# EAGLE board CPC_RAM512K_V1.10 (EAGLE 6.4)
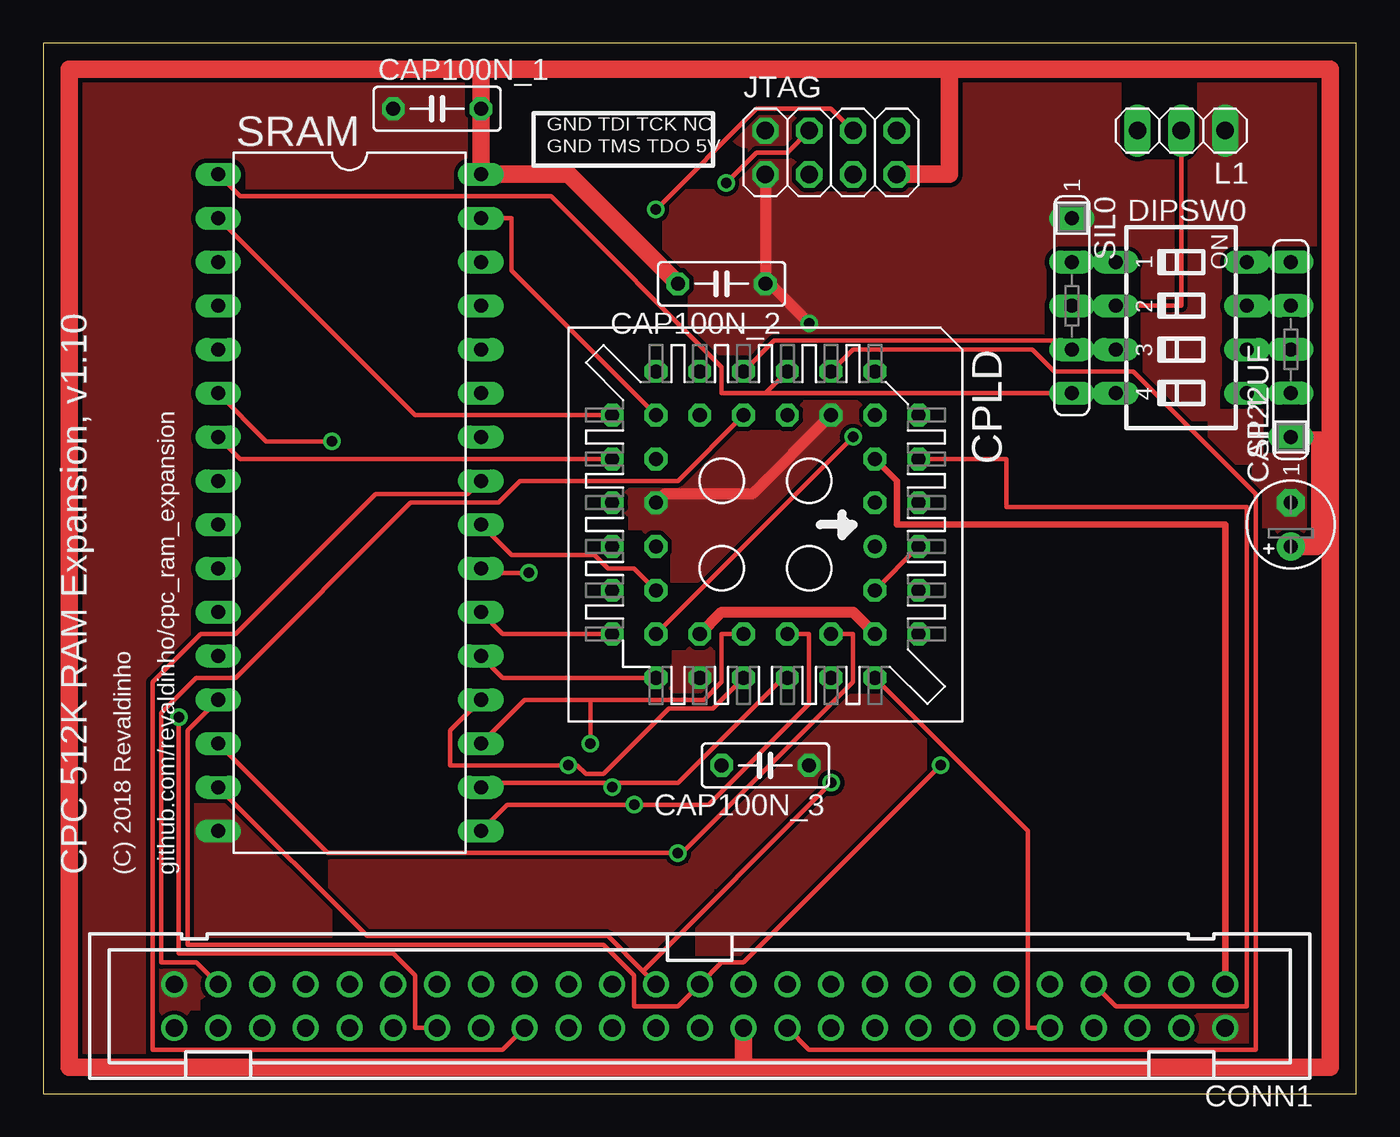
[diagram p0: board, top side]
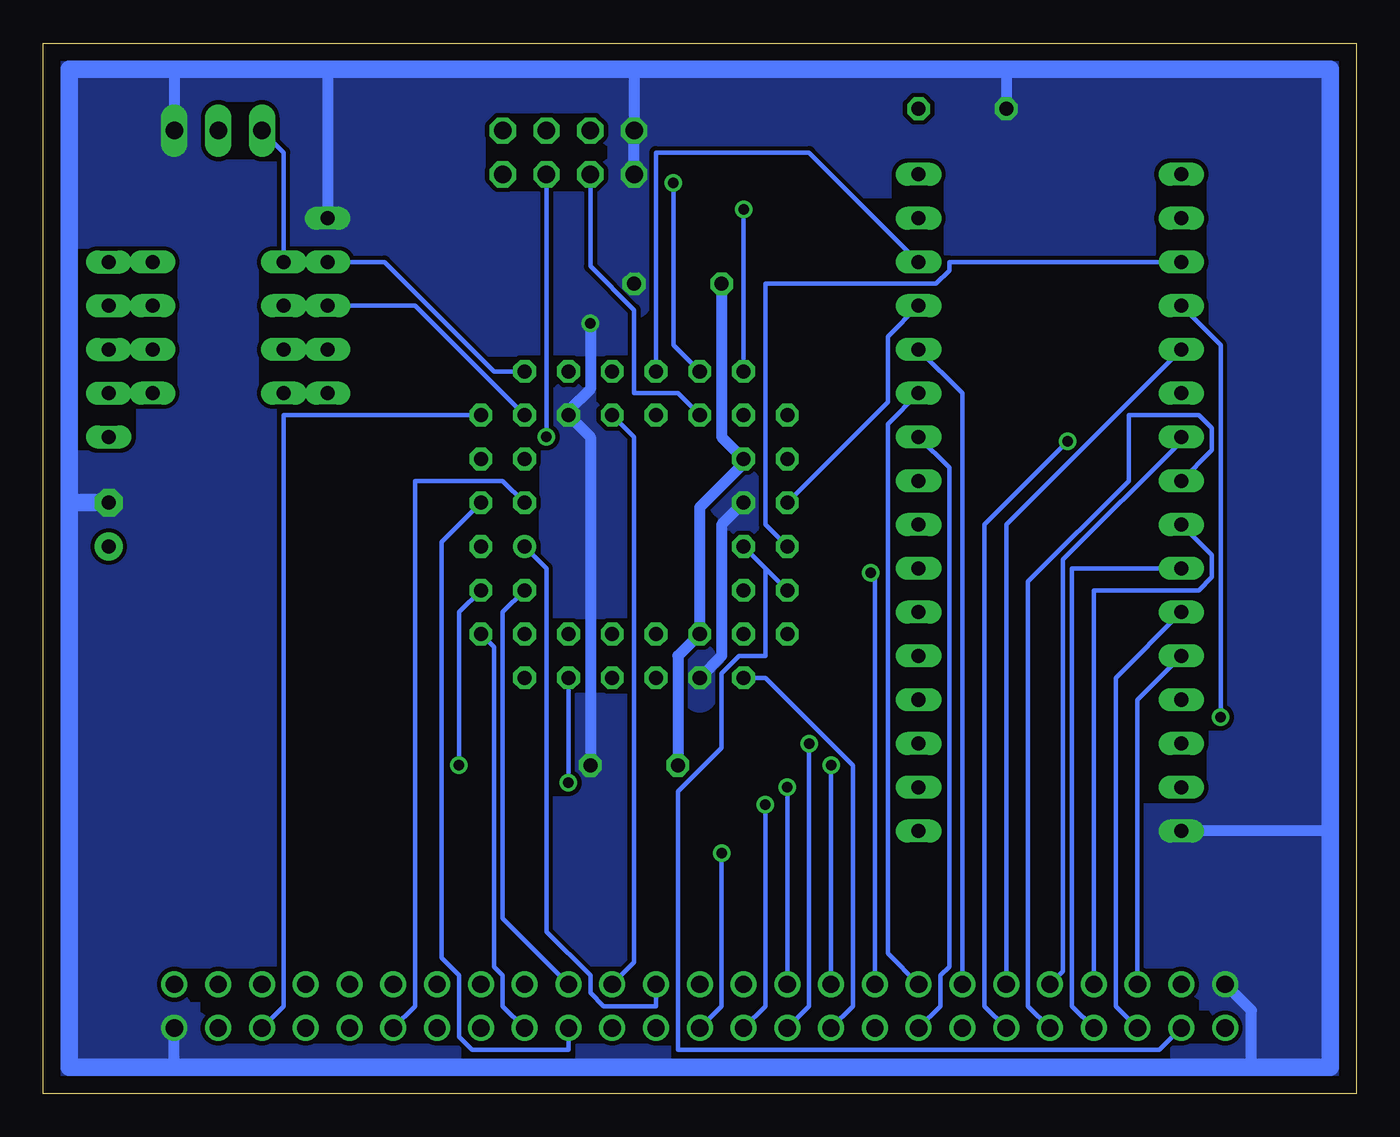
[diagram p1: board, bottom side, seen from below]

Size 76.2 x 60.96 mm. Coordinates in mm from the lower left corner, seen from the top.
Outline: 0,0 76.2,0 76.2,60.96 0,60.96 0,0
Copper layers (1*16): Top 0.035mm / dielectric 1.5mm / Bottom 0.035mm
Design rules "default": minimum track width 10mil, minimum drill 24mil, track to track 8mil, track to pad 8mil, pad to pad 8mil, via to via 8mil, smd to smd 8mil, copper to edge 40mil, drill to drill 8mil, minimum pad ring 10mil, minimum via ring 8mil, stop-mask expansion 4mil, vias tented up to drill 0mil, thermal gap 10mil
Net classes: 0 signal: width 0.254 mm, clearance 0.254 mm; 1 supply: width 0.635 mm, clearance 0.254 mm

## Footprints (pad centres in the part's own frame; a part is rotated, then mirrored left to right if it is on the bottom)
E2,5-5 = drill 0.813 pad 1.6: + -1.27,0 | drill 0.813 pad 1.6 octagon: - 1.27,0
C050-025X075 = drill 0.813 octagon: 1 -2.54,0; 2 2.54,0
PAK100/2500-50 = drill 1 pad 1.422: 1 -30.48,-1.27; 2 -30.48,1.27; 3 -27.94,-1.27; 4 -27.94,1.27; 5 -25.4,-1.27; 6 -25.4,1.27; 7 -22.86,-1.27; 8 -22.86,1.27; 9 -20.32,-1.27; 10 -20.32,1.27; 11 -17.78,-1.27; 12 -17.78,1.27; 13 -15.24,-1.27; 14 -15.24,1.27; 15 -12.7,-1.27; 16 -12.7,1.27; 17 -10.16,-1.27; 18 -10.16,1.27; 19 -7.62,-1.27; 20 -7.62,1.27; 21 -5.08,-1.27; 22 -5.08,1.27; 23 -2.54,-1.27; 24 -2.54,1.27; 25 0,-1.27; 26 0,1.27; 27 2.54,-1.27; 28 2.54,1.27; 29 5.08,-1.27; 30 5.08,1.27; 31 7.62,-1.27; 32 7.62,1.27; 33 10.16,-1.27; 34 10.16,1.27; 35 12.7,-1.27; 36 12.7,1.27; 37 15.24,-1.27; 38 15.24,1.27; 39 17.78,-1.27; 40 17.78,1.27; 41 20.32,-1.27; 42 20.32,1.27; 43 22.86,-1.27; 44 22.86,1.27; 45 25.4,-1.27; 46 25.4,1.27; 47 27.94,-1.27; 48 27.94,1.27; 49 30.48,-1.27; 50 30.48,1.27
PLCC-S44-SOCKET = drill 0.813: 1 1.27,6.35 | drill 0.813 octagon: 2 -1.27,8.89; 3 -1.27,6.35; 4 -3.81,8.89; 5 -3.81,6.35; 6 -6.35,8.89; 7 -8.89,6.35; 8 -6.35,6.35; 9 -8.89,3.81; 10 -6.35,3.81; 11 -8.89,1.27; 12 -6.35,1.27; 13 -8.89,-1.27; 14 -6.35,-1.27; 15 -8.89,-3.81; 16 -6.35,-3.81; 17 -8.89,-6.35; 18 -6.35,-8.89; 19 -6.35,-6.35; 20 -3.81,-8.89; 21 -3.81,-6.35; 22 -1.27,-8.89; 23 -1.27,-6.35; 24 1.27,-8.89; 25 1.27,-6.35; 26 3.81,-8.89; 27 3.81,-6.35; 28 6.35,-8.89; 29 8.89,-6.35; 30 6.35,-6.35; 31 8.89,-3.81; 32 6.35,-3.81; 33 8.89,-1.27; 34 6.35,-1.27; 35 8.89,1.27; 36 6.35,1.27; 37 8.89,3.81; 38 6.35,3.81; 39 8.89,6.35; 40 6.35,8.89; 41 6.35,6.35; 42 3.81,8.89; 43 3.81,6.35; 44 1.27,8.89
SD4-04 = drill 0.813 long: 1 -3.81,-3.81; 2 -1.27,-3.81; 3 1.27,-3.81; 4 3.81,-3.81; 5 3.81,3.81; 6 1.27,3.81; 7 -1.27,3.81; 8 -3.81,3.81
2X04 = drill 1.016 octagon: 1 -3.81,-1.27; 2 -3.81,1.27; 3 -1.27,-1.27; 4 -1.27,1.27; 5 1.27,-1.27; 6 1.27,1.27; 7 3.81,-1.27; 8 3.81,1.27
1X03 = drill 1.016 long: 1 -2.54,0; 2 0,0; 3 2.54,0
SIL5 = drill 0.813 long: 1 -5.08,0; 2 -2.54,0; 3 0,0; 4 2.54,0; 5 5.08,0
DIL32 = drill 0.813 long: 1 -19.05,-7.62; 2 -16.51,-7.62; 3 -13.97,-7.62; 4 -11.43,-7.62; 5 -8.89,-7.62; 6 -6.35,-7.62; 7 -3.81,-7.62; 8 -1.27,-7.62; 9 1.27,-7.62; 10 3.81,-7.62; 11 6.35,-7.62; 12 8.89,-7.62; 13 11.43,-7.62; 14 13.97,-7.62; 15 16.51,-7.62; 16 19.05,-7.62; 17 19.05,7.62; 18 16.51,7.62; 19 13.97,7.62; 20 11.43,7.62; 21 8.89,7.62; 22 6.35,7.62; 23 3.81,7.62; 24 1.27,7.62; 25 -1.27,7.62; 26 -3.81,7.62; 27 -6.35,7.62; 28 -8.89,7.62; 29 -11.43,7.62; 30 -13.97,7.62; 31 -16.51,7.62; 32 -19.05,7.62

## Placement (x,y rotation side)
CAP22UF  [E2,5-5]  72.39,33.02 90 top
CAP100N_1  [C050-025X075]  22.86,57.15 0 top
CAP100N_2  [C050-025X075]  39.37,46.99 180 top
CAP100N_3  [C050-025X075]  41.91,19.05 180 top
CONN1  [PAK100/2500-50]  38.1,5.08 180 top
CPLD  [PLCC-S44-SOCKET]  41.91,33.02 270 top
DIPSW0  [SD4-04]  66.04,44.45 270 top
JTAG  [2X04]  45.72,54.61 0 top
L1  [1X03]  66.04,55.88 180 top
SIL0  [SIL5]  59.69,45.72 270 top
SIL1  [SIL5]  72.39,43.18 90 top
SRAM  [DIL32]  17.78,34.29 270 top

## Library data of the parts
CAP22UF CAP100N_1-CAP100N_3 = resistor
CONN1 = con-3m
CPLD SRAM = ic-package
DIPSW0 = switch-dil
JTAG L1 = pinhead
SIL0 SIL1 = resistor-sil

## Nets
A0: CONN1.33 SRAM.23
A1: CONN1.34 SRAM.25
A2: CONN1.35 SRAM.27
A3: CONN1.36 SRAM.26
A4: CONN1.37 SRAM.28
A5: CONN1.38 SRAM.4
A6: CONN1.39 SRAM.5
A7: CONN1.40 SRAM.6
A8: CONN1.41 CPLD.20 SRAM.7
A9: CONN1.42 SRAM.8
A10: CONN1.43 SRAM.9
A11: CONN1.44 SRAM.10
A12: CONN1.45 SRAM.12
A13: CONN1.46 SRAM.11
A14: CONN1.47 CPLD.14
A15: CONN1.48 CPLD.25 CPLD.26
BUSACK_B: CONN1.13
BUSRESET_B: CONN1.11
BUSRQ_B: CONN1.14
CLK: CONN1.1 CPLD.5
CURSOR: CONN1.5
D0: CONN1.25 CPLD.42 SRAM.13
D1: CONN1.26 CPLD.38 SRAM.14
D2: CONN1.27 CPLD.37 SRAM.15
D3: CONN1.28 CPLD.36 SRAM.17
D4: CONN1.29 CPLD.35 SRAM.18
D5: CONN1.30 CPLD.34 SRAM.19
D6: CONN1.31 CPLD.33 SRAM.20
D7: CONN1.32 CPLD.29 SRAM.21
DIP0: CPLD.7 DIPSW0.1 L1.3 SIL0.2
DIP0_PU: DIPSW0.8 SIL1.5
DIP1: CPLD.8 DIPSW0.2 L1.2 SIL0.3
DIP1_PU: DIPSW0.7 SIL1.4
DIP2_PU: DIPSW0.6 SIL1.3
DIP3_PU: DIPSW0.5 SIL1.2
EXP_B: CONN1.3
HALT_B: CONN1.17
HIADR0: CPLD.24 SRAM.3
HIADR1: CPLD.19 SRAM.31
HIADR2: CPLD.18 SRAM.2
HIADR3: CPLD.13 DIPSW0.3 SIL0.4 SRAM.30
HIADR4: CPLD.11 DIPSW0.4 SIL0.5 SRAM.1
INT_B: CONN1.16
IOREQ_B: CONN1.20 CPLD.2
LPEN: CONN1.4
M1_B: CONN1.22 CPLD.9
MREQ_B: CONN1.23 CPLD.1
NMI_B: CONN1.15
RAMCS_B: CPLD.28 SRAM.22
RAMDIS: CONN1.6 CPLD.6
RAMOE_B: CPLD.27 SRAM.24
RAMRD_B: CONN1.7 CPLD.4
RAMWE_B: CPLD.22 SRAM.29
RD_B: CONN1.19 CPLD.43 CPLD.44
READY: CONN1.12 CPLD.3
RESET_B: CONN1.10 CPLD.39
RFSH_B: CONN1.21 CPLD.12
ROMDIS: CONN1.8
ROMEN_B: CONN1.9
SOUND: CONN1.50
TCK: CPLD.17 JTAG.6
TDI: CPLD.15 JTAG.4
TDO: CPLD.30 JTAG.5
TMS: CPLD.16 JTAG.3
VDD [supply]: CAP22UF.+ CAP100N_1.2 CAP100N_2.2 CAP100N_3.2 CONN1.24 CPLD.21 CPLD.32 CPLD.41 JTAG.7 SIL1.1 SRAM.32
VSS [supply]: CAP22UF.- CAP100N_1.1 CAP100N_2.1 CAP100N_3.1 CONN1.2 CONN1.49 CPLD.10 CPLD.23 CPLD.31 JTAG.1 JTAG.2 L1.1 SIL0.1 SRAM.16
WR_B: CONN1.18 CPLD.40

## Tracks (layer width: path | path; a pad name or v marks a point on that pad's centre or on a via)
A0  (via drill 0.61)
  Top 0.254: SRAM.23 25.65,30.23 v28.19,30.23
  Bottom 0.254: v28.19,30.23 27.94,29.97 CONN1.33
A1
  Top 0.254: SRAM.25 24.64,34.8 19.3,34.8 11.18,26.67 9.14,26.67 6.35,23.88 6.35,2.54 26.67,2.54 CONN1.34
A2
  Bottom 0.254: SRAM.27 27.18,38.86 27.18,8.13 CONN1.35
A3
  Bottom 0.254: SRAM.26 23.62,36.32 23.62,7.37 24.13,6.86 24.13,5.08 CONN1.36
A4
  Bottom 0.254: SRAM.28 22.86,40.64 CONN1.37
A5  (via drill 0.61)
  Top 0.254: v7.87,21.84 7.87,8.13 20.32,8.13 21.59,6.86 21.59,3.81 CONN1.38
  Bottom 0.254: SRAM.4 7.87,43.43 v7.87,21.84
A6
  Bottom 0.254: SRAM.5 20.32,33.02 CONN1.39
A7  (via drill 0.61)
  Top 0.254: SRAM.6 12.95,37.85 v16.76,37.85
  Bottom 0.254: v16.76,37.85 21.59,33.02 21.59,5.08 CONN1.40
A8
  Top 0.254: SRAM.7 11.43,36.83 CPLD.20
  Bottom 0.254: CONN1.41 17.02,7.11 17.02,30.99 10.16,37.85 SRAM.7
A9
  Bottom 0.254: SRAM.8 8.38,37.34 8.38,38.61 9.14,39.37 13.21,39.37 13.21,35.56 19.05,29.72 19.05,5.08 CONN1.42
A10
  Bottom 0.254: SRAM.9 8.38,31.24 8.38,29.97 9.14,29.21 15.24,29.21 CONN1.43
A11
  Bottom 0.254: SRAM.10 16.51,30.48 16.51,5.08 CONN1.44
A12
  Bottom 0.254: SRAM.12 12.7,22.86 CONN1.45
A13
  Bottom 0.254: SRAM.11 13.97,24.13 13.97,5.08 CONN1.46
A14
  Top 0.254: CPLD.14 36.83,35.56 27.69,35.56 26.42,34.29 21.34,34.29 11.18,24.13 8.89,24.13 6.86,22.1 6.86,7.62 8.89,7.62 CONN1.47
A15
  Bottom 0.254: CPLD.25 34.29,30.48 | 34.29,30.48 CPLD.26 | CONN1.48 11.43,2.54 39.37,2.54 39.37,17.53 36.83,20.07 36.83,24.38 35.81,25.4 34.29,25.4 34.29,30.48
CLK
  Top 0.381: CPLD.5 49.53,35.56 49.53,33.02 68.58,33.02 CONN1.1
D0  (via drill 0.61)
  Top 0.254: SRAM.13 8.38,21.08 8.38,8.64 32.51,8.64 34.29,6.86 34.29,5.08 36.83,5.08 CONN1.25 39.37,7.62 40.64,7.62 v52.07,19.05
  Bottom 0.254: CPLD.42 52.07,27.94 v52.07,19.05
D1  (via drill 0.61)
  Top 0.254: SRAM.14 16.51,13.97 v36.83,13.97 37.08,13.97 46.99,23.88 46.99,26.67 CPLD.38
  Bottom 0.254: CONN1.26 36.83,5.08 v36.83,13.97
D2  (via drill 0.61)
  Top 0.254: SRAM.15 18.8,9.14 32.77,9.14 34.8,7.11 | CONN1.27 34.8,7.11 | 34.8,7.11 v45.72,18.03
  Bottom 0.254: v45.72,18.03 CPLD.37
D3  (via drill 0.61)
  Top 0.254: SRAM.17 26.92,16.76 v34.29,16.76 38.61,16.76 44.45,22.61 44.45,26.67 CPLD.36
  Bottom 0.254: CONN1.28 34.29,5.08 v34.29,16.76
D4  (via drill 0.61)
  Top 0.254: SRAM.18 25.65,18.03 33.02,18.03 | 33.02,18.03 36.83,18.03 42.93,24.13 CPLD.35 | 33.02,18.03 v33.02,17.78
  Bottom 0.254: v33.02,17.78 CONN1.29
D5  (via drill 0.61)
  Top 0.254: SRAM.19 27.94,22.86 31.75,22.86 | 31.75,22.86 38.35,22.86 39.37,23.88 39.37,26.67 CPLD.34 | 31.75,22.86 v31.75,20.32
  Bottom 0.254: CONN1.30 31.75,5.08 v31.75,20.32
D6  (via drill 0.61)
  Top 0.254: SRAM.20 23.62,21.08 23.62,19.05 v30.48,19.05 30.99,19.05 31.5,18.54 32.51,18.54 36.32,22.35 38.86,22.35 CPLD.33
  Bottom 0.254: v30.48,19.05 CONN1.31
D7
  Top 0.254: SRAM.21 26.67,24.13 CPLD.29
  Bottom 0.254: CONN1.32 29.21,5.08 29.21,19.05 34.29,24.13 CPLD.29
DIP0
  Top 0.254: SIL0.2 DIPSW0.1
  Bottom 0.254: CPLD.7 50.04,41.91 56.39,48.26 SIL0.2 | L1.3 62.23,54.61 DIPSW0.1
DIP0_PU
  Top 0.254: SIL1.5 DIPSW0.8
DIP1
  Top 0.254: SIL0.3 DIPSW0.2 66.04,45.72 L1.2
  Bottom 0.254: CPLD.8 54.61,45.72 SIL0.3
DIP1_PU
  Top 0.254: SIL1.4 DIPSW0.7
DIP2_PU
  Top 0.254: SIL1.3 DIPSW0.6
DIP3_PU
  Top 0.254: SIL1.2 DIPSW0.5
HIADR0
  Bottom 0.254: SRAM.3 23.62,48.26 23.62,47.75 24.38,46.99 34.29,46.99 34.29,33.02 CPLD.24
HIADR1
  Top 0.254: CPLD.19 27.18,47.75 27.18,50.8 SRAM.31
HIADR2
  Top 0.254: SRAM.2 21.59,39.37 CPLD.18
HIADR3
  Top 0.254: DIPSW0.3 SIL0.4 59.18,43.69 42.42,43.69 CPLD.13
  Bottom 0.254: SRAM.30 31.75,54.61 40.64,54.61 CPLD.13
HIADR4
  Top 0.254: DIPSW0.4 SIL0.5 41.91,40.64 | SRAM.1 11.43,52.07 29.46,52.07 39.37,42.16 39.37,40.64 41.91,40.64 | CPLD.11 41.91,40.64
IOREQ_B
  Bottom 0.254: CPLD.2 53.09,32 53.09,7.87 52.07,6.86 52.07,3.3 51.31,2.54 45.72,2.54 CONN1.20
M1_B
  Top 0.254: CPLD.9 46.99,43.18 57.4,43.18 58.67,41.91 63.25,41.91 70.36,34.8 70.36,2.54 44.45,2.54 CONN1.22
MREQ_B
  Bottom 0.254: CPLD.1 46.99,30.48 46.99,9.4 44.45,6.86 44.45,5.84 43.69,5.08 40.64,5.08 CONN1.23
RAMCS_B
  Top 0.254: SRAM.22 26.67,26.67 CPLD.28
RAMDIS
  Bottom 0.254: CPLD.6 62.23,39.37 62.23,5.08 CONN1.6
RAMOE_B
  Top 0.254: SRAM.24 27.18,31.24 32,31.24 32.77,30.48 34.29,30.48 CPLD.27
RAMRD_B
  Top 0.254: CPLD.4 55.88,36.83 55.88,34.04 69.85,34.04 69.85,5.08 62.23,5.08 CONN1.7
RAMWE_B
  Bottom 0.254: CPLD.22 27.18,40.13 27.18,43.94 SRAM.29
RD_B
  Top 0.254: CPLD.44 CPLD.43
  Bottom 0.254: CONN1.19 49.53,10.16 49.53,27.94 CPLD.43
READY
  Bottom 0.254: CPLD.3 49.53,35.56 54.61,35.56 54.61,5.08 CONN1.12
RESET_B
  Top 0.254: CPLD.39 57.15,15.24 57.15,3.81 CONN1.10
RFSH_B
  Bottom 0.254: CPLD.12 41.91,38.1 41.91,7.62 CONN1.21
TCK  (via drill 0.61)
  Top 0.254: v35.56,51.31 41.4,57.15 45.72,57.15 JTAG.6
  Bottom 0.254: v35.56,51.31 CPLD.17
TDI  (via drill 0.61)
  Top 0.254: v39.62,52.83 41.4,54.61 43.18,54.61 JTAG.4
  Bottom 0.254: CPLD.15 39.62,43.43 v39.62,52.83
TDO  (via drill 0.61)
  Top 0.254: v46.99,38.1 CPLD.30
  Bottom 0.254: JTAG.5 v46.99,38.1
TMS
  Bottom 0.254: CPLD.16 39.37,40.64 41.91,40.64 41.91,45.47 44.45,48.01 JTAG.3
VDD
  Top 0.635: CPLD.41 46.99,27.94 39.37,27.94 CPLD.32 | 74.68,38.1 73.91,38.1 | 73.91,38.1 SIL1.1 | 73.91,31.75 73.91,38.1
  Top 1.016: 40.64,1.52 1.52,1.52 1.52,59.44 25.4,59.44 | 40.64,1.52 74.68,1.52 74.68,38.1 74.68,59.44 55.37,59.44 52.58,59.44 | 52.58,59.44 25.4,59.44 | CAP22UF.+ 73.91,31.75 | 40.64,1.52 CONN1.24 | 52.58,59.44 52.58,53.34 JTAG.7 | 25.4,59.44 CAP100N_1.2 SRAM.32 30.48,53.34 CAP100N_2.2
  Bottom 0.635: CAP100N_2.2 36.83,38.1 CPLD.21 35.56,36.58 38.1,34.04 CPLD.32 39.37,25.4 CAP100N_3.2
VSS  (via drill 0.61)
  Top 0.635: CPLD.23 36.07,34.8 41.15,34.8 CPLD.10 | JTAG.1 CAP100N_2.1 42.16,46.99 v44.45,44.7
  Bottom 0.635: CPLD.31 36.83,25.4 36.83,33.02 CPLD.23 | CAP100N_3.1 44.45,38.1 CPLD.10 45.72,39.62 44.45,40.89 v44.45,44.7 | JTAG.1 JTAG.2 41.91,59.44 | 1.52,15.24 SRAM.16 | 59.69,59.44 SIL0.1 | 20.32,59.44 CAP100N_1.1 | 68.58,1.52 CONN1.2 | CONN1.49 6.1,4.83 6.1,1.52 | 68.58,59.44 L1.1
  Bottom 1.016: 74.68,34.29 74.68,1.52 68.58,1.52 6.1,1.52 1.52,1.52 1.52,15.24 1.52,59.44 20.32,59.44 41.91,59.44 59.69,59.44 68.58,59.44 74.68,59.44 74.68,34.29 | 74.68,34.29 CAP22UF.-
  pour Top: 0,0 0,59.69 76.2,59.69 76.2,0
  pour Bottom: 0,0 0,59.69 76.2,59.69 76.2,0
WR_B
  Bottom 0.254: CPLD.40 50.04,25.91 50.04,7.37 49.53,6.86 49.53,5.08 CONN1.18

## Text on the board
tPlace: GND TDI TCK NC | GND TMS TDO 5V | CPC 512K RAM Expansion, v1.10 | (C) 2018 Revaldinho | github.com/revaldinho/cpc_ram_expansion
